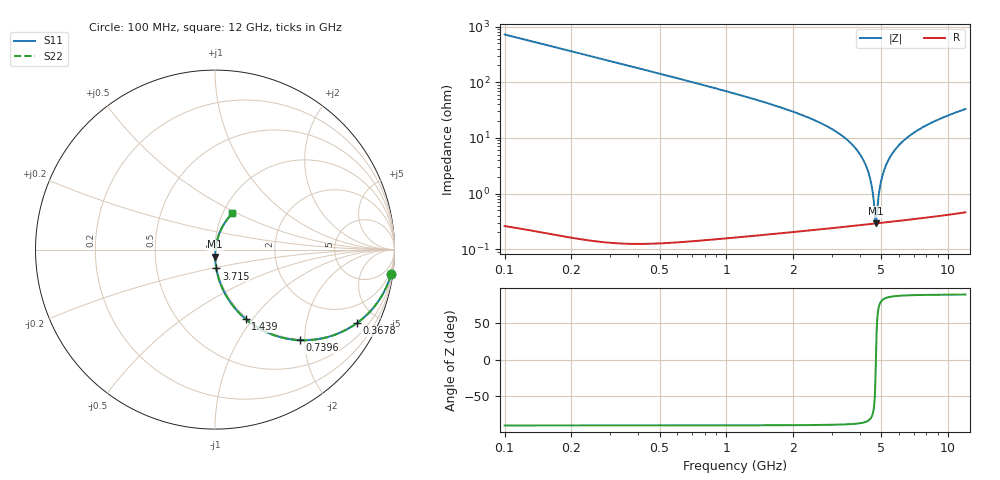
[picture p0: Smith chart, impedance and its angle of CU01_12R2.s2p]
! S-parameter model data by Modelithics Inc. support@modelithics.com 813-866-6335 Tampa FL USA
! S-Parameter data specifications:
! Substrate: 20-mil Rogers, substrate thickness, H=0.508mm, Dielectric constant, Er=3.75
! PCB Mounting Pad Footprint: Pad width, PadW=0.35mm , Pad length, PadL=0.30mm , Pad gap, PadG (edge-to-edge)=0.25mm , Reference planes=0.85mm apart
! Created Tue May  8 14:01:25 2018
# hz S ma R 50
! 2 Port Network Data from SP1.SP block
! freq  magS11  angS11  magS21  angS21  magS12  angS12  magS22  angS22
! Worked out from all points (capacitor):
!   801 points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, 100 MHz to 12 GHz, reference 50 ohm
!   read as one part in series: C = 2.21 pF near 159.5 MHz
!   lowest |Z| = 292 mohm at 4.741 GHz (marker M1)
!   series resonance near 4.735 GHz, so ESL is about 510 pH
!   S11 on the Smith chart (normalised r, x): 100 MHz: 1, -14; 367.8 MHz: 0.98, -3.85; 739.6 MHz: 0.98, -1.89; 1.439 GHz: 0.98, -0.92; 3.715 GHz: 0.99, -0.21; 12 GHz: 1.11, +0.47
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1e8  0.9904 -8.0  0.1377 82.0  0.1377 82.0  0.9904 -8.0
2.33875e8  0.9507 -18.3  0.3095 71.7  0.3095 71.7  0.9507 -18.3
3.6775e8  0.8894 -27.5  0.4565 62.4  0.4565 62.4  0.8894 -27.5
7.39625e8  0.6904 -47.0  0.7224 42.9  0.7224 42.9  0.6904 -47.0
1.052e9  0.5499 -57.5  0.8339 32.3  0.8339 32.3  0.5499 -57.5
1.43875e9  0.4221 -66.2  0.9049 23.6  0.9049 23.6  0.4221 -66.2
2.09325e9  0.282 -75.2  0.9574 14.4  0.9574 14.4  0.282 -75.2
3.714625e9  0.1053 -86.2  0.9918 2.4  0.9918 2.4  0.1053 -86.2
4.071625e9  0.08025 -87.4  0.994 0.7  0.994 0.7  0.08025 -87.4
4.741e9  0.03972 -88.2  0.9963 -2.3  0.9963 -2.3  0.03972 -88.2
5.18725e9  0.01625 -83.6  0.9968 -4.1  0.9968 -4.1  0.01625 -83.6
5.30625e9  0.01047 -77.9  0.9969 -4.6  0.9969 -4.6  0.01047 -77.9
5.469875e9  0.003682 -39.4  0.9969 -5.2  0.9969 -5.2  0.003682 -39.4
5.5145e9  0.003058 -4.2  0.9969 -5.3  0.9969 -5.3  0.003058 -4.2
5.559125e9  0.00376 29.8  0.9968 -5.5  0.9968 -5.5  0.00376 29.8
5.767375e9  0.01223 69.0  0.9967 -6.3  0.9967 -6.3  0.01223 69.0
6.05e9  0.02462 75.3  0.9964 -7.3  0.9964 -7.3  0.02462 75.3
6.362375e9  0.03788 76.7  0.9959 -8.3  0.9959 -8.3  0.03788 76.7
6.79375e9  0.05535 76.8  0.995 -9.7  0.995 -9.7  0.05535 76.8
8.04325e9  0.1016 74.3  0.9911 -13.6  0.9911 -13.6  0.1016 74.3
1.002162e10  0.1663 69.4  0.9819 -19.3  0.9819 -19.3  0.1663 69.4
1.2e10  0.2246 64.3  0.9699 -24.6  0.9699 -24.6  0.2246 64.3
